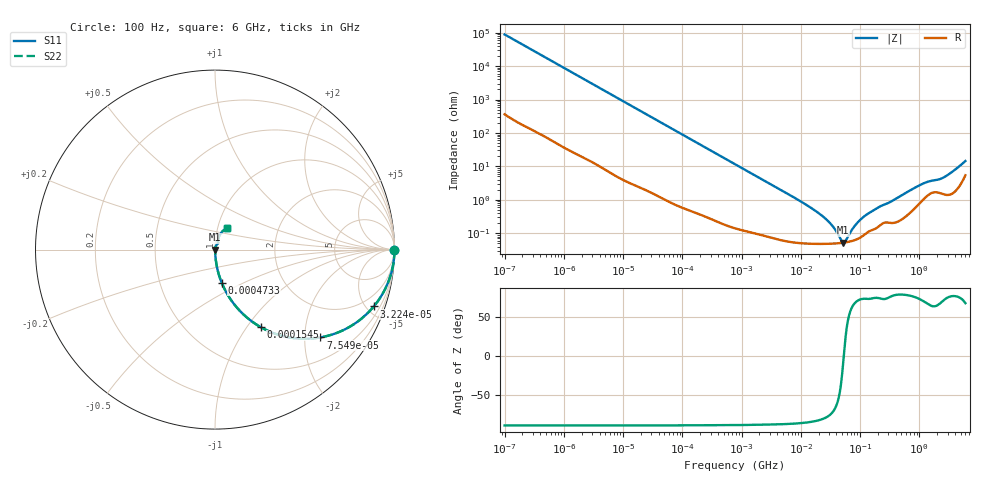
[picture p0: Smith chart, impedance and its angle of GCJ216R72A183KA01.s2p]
!Murata Part Number: GCJ216R72A183KA01
!These Parameters are Measured in Series Mode Connection
!Data Generated on Mar 13, 2026
!  o--ll--o
!Port1  Port2
!  o------o
!Operation Temp=25[degC], DC Bias Voltage=0[V]
!Freq. Start=100[Hz] Stop=6[GHz] 401[Steps]
# Hz S RI R 50
!Freq.(Hz) S11(Real) S11(Imag) S21(Real) S21(Imag) S12(Real) S12(Imag) S22(Real) S22(Imag)
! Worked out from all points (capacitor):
!   401 points, 100 Hz to 6 GHz, reference 50 ohm
!   read as one part in series: C = 18 nF near 109 Hz
!   lowest |Z| = 52.6 mohm at 52.11 MHz (marker M1)
!   series resonance near 53.16 MHz, so ESL is about 500 pH
!   S11 on the Smith chart (normalised r, x): 100 Hz: open; 32.24 kHz: 1.03, -5.57; 75.5 kHz: 1.01, -2.39; 154.5 kHz: 1.01, -1.17; 473.3 kHz: 1.00, -0.38; 6 GHz: 1.11, +0.27
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100  1 -0.00113  5.9e-06 0.00113  5.9e-06 0.00113  1 -0.00113
2008  0.9994 -0.0225  0.000606 0.0225  0.000606 0.0225  0.9994 -0.0225
10066  0.987 -0.1109  0.013 0.1109  0.013 0.1109  0.987 -0.1109
32244  0.8846 -0.3168  0.1154 0.3168  0.1154 0.3168  0.8846 -0.3168
40335  0.8311 -0.3719  0.1689 0.3719  0.1689 0.3719  0.8311 -0.3719
75495  0.587 -0.4894  0.413 0.4894  0.413 0.4894  0.587 -0.4894
154540  0.2562 -0.4329  0.7438 0.4329  0.7438 0.4329  0.2562 -0.4329
252896  0.1157 -0.3156  0.8843 0.3156  0.8843 0.3156  0.1157 -0.3156
473344  0.0372 -0.1844  0.9628 0.1844  0.9628 0.1844  0.0372 -0.1844
774597  0.015 -0.1155  0.985 0.1155  0.985 0.1155  0.015 -0.1155
2481164  0.00218 -0.0368  0.9978 0.0368  0.9978 0.0368  0.00218 -0.0368
1.555665e7  0.000513 -0.00543  0.9995 0.00543  0.9995 0.00543  0.000513 -0.00543
3.045065e7  0.000489 -0.00204  0.9995 0.00204  0.9995 0.00204  0.000489 -0.00204
5.211241e7  0.000521 -6.86e-05  0.9995 6.86e-05  0.9995 6.86e-05  0.000521 -6.86e-05
5.699437e7  0.000534 0.000245  0.9995 -0.000245  0.9995 -0.000245  0.000534 0.000245
7.797396e7  0.000609 0.00138  0.9994 -0.00138  0.9994 -0.00138  0.000609 0.00138
1.115611e8  0.000842 0.00284  0.9992 -0.00284  0.9992 -0.00284  0.000842 0.00284
1.996653e8  0.00156 0.0056  0.9984 -0.0056  0.9984 -0.0056  0.00156 0.0056
3.124326e8  0.00212 0.00804  0.9979 -0.00804  0.9979 -0.00804  0.00212 0.00804
1.094528e9  0.00974 0.0273  0.9903 -0.0273  0.9903 -0.0273  0.00974 0.0273
2.562649e9  0.0163 0.0427  0.9837 -0.0427  0.9837 -0.0427  0.0163 0.0427
6e9  0.0668 0.1192  0.9332 -0.1192  0.9332 -0.1192  0.0668 0.1192
